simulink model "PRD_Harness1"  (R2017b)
settings: Solver=FixedStepDiscrete  StartTime=0.0  StopTime=4  FixedStep=0.01  RelTol=1e-3  EnableMultiTasking=on
undefined symbols (not defined in the file): sigbuilder_block

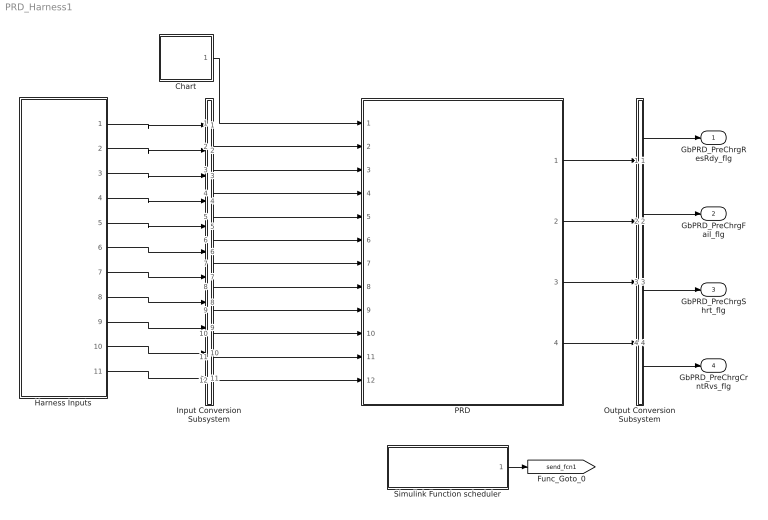
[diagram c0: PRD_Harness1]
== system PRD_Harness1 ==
  Chart : Stateflow chart  TreatAsAtomicUnit=on
  Harness Inputs : Subsystem  Tag=STV Subsys  LoadFcn=sigbuilder_block('load');  StartFcn=sigbuilder_block('start');  StopFcn=sigbuilder_block('stop');  ClipboardFcn=sigbuilder_block('clipboard');  mask(Sigbuilder block){tuvar=[0:10]}
      mask init:
      | if ~strcmp(get_param(bdroot(gcb),'SimulationStatus'),'stopped'),tuvar = sigbuilder_block('maskInit'); end
  Input Conversion Subsystem : Subsystem  Tag=__SLT_ICS__  Description=Signal spec. and routing
  Output Conversion Subsystem : Subsystem  Tag=__SLT_OCS__  Description=Signal spec. and routing
  PRD : ModelReference  ModelNameDialog=PRD  SimulationMode=Normal  ModelReferenceVersion='M101C101R103'
  Simulink Function scheduler : Test Sequence  Tag=__SLT_FCN_CALL__  TreatAsAtomicUnit=on
  GbPRD_PreChrgResRdy_flg : Outport  OutDataTypeStr=boolean  PortDimensions=[1]
  GbPRD_PreChrgFail_flg : Outport  Port=2  OutDataTypeStr=boolean  PortDimensions=[1]
  GbPRD_PreChrgShrt_flg : Outport  Port=3  OutDataTypeStr=boolean  PortDimensions=[1]
  GbPRD_PreChrgCrntRvs_flg : Outport  Port=4  OutDataTypeStr=boolean  PortDimensions=[1]
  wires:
  Harness Inputs/1(GeCTC_CtrCtlState_enum) -> Input Conversion Subsystem/1(Inport_1)
  Harness Inputs/2(GbCTC_PreChrgTimeOutFlt_flg) -> Input Conversion Subsystem/2(Inport_2)
  Harness Inputs/3(GcHDP_PackCrnt_A) -> Input Conversion Subsystem/3(Inport_3)
  Harness Inputs/4(GbHDP_PackCrntVld_flg) -> Input Conversion Subsystem/4(Inport_4)
  Harness Inputs/5(GbHDP_PackVoltVld_flg) -> Input Conversion Subsystem/5(Inport_5)
  Harness Inputs/6(GcHDP_PackVolt_V) -> Input Conversion Subsystem/6(Inport_6)
  Harness Inputs/7(GcHDP_PosCtlVolt_V) -> Input Conversion Subsystem/7(Inport_7)
  Harness Inputs/8(GbHDP_PosCtlVoltVld_flg) -> Input Conversion Subsystem/8(Inport_8)
  Harness Inputs/9(GcCDP_SumCellVolt_V) -> Input Conversion Subsystem/9(Inport_9)
  Harness Inputs/10(GbCDP_SumCellVoltVld_flg) -> Input Conversion Subsystem/10(Inport_10)
  Harness Inputs/11(GcRTC_ShelveTime_min) -> Input Conversion Subsystem/11(Inport_11)
  Output Conversion Subsystem/1(Outport_1) -> GbPRD_PreChrgResRdy_flg/1
  Output Conversion Subsystem/2(Outport_2) -> GbPRD_PreChrgFail_flg/1
  Output Conversion Subsystem/3(Outport_3) -> GbPRD_PreChrgShrt_flg/1
  Output Conversion Subsystem/4(Outport_4) -> GbPRD_PreChrgCrntRvs_flg/1
  Chart/1(RUN10ms()) -> PRD/1
  Input Conversion Subsystem/2(Outport_2) -> PRD/2
  Input Conversion Subsystem/3(Outport_3) -> PRD/3
  Input Conversion Subsystem/4(Outport_4) -> PRD/4
  Input Conversion Subsystem/5(Outport_5) -> PRD/5
  Input Conversion Subsystem/6(Outport_6) -> PRD/6
  Input Conversion Subsystem/7(Outport_7) -> PRD/7
  Input Conversion Subsystem/8(Outport_8) -> PRD/8
  Input Conversion Subsystem/9(Outport_9) -> PRD/9
  Input Conversion Subsystem/10(Outport_10) -> PRD/10
  Input Conversion Subsystem/11(Outport_11) -> PRD/11
  Input Conversion Subsystem/12(Outport_12) -> PRD/12
  PRD/1 -> Output Conversion Subsystem/1(Inport_1)
  PRD/2 -> Output Conversion Subsystem/2(Inport_2)
  PRD/3 -> Output Conversion Subsystem/3(Inport_3)
  PRD/4 -> Output Conversion Subsystem/4(Inport_4)
  Simulink Function scheduler/1(PRD_PreChrgResDiag_10ms()) -> [send_fcn1]

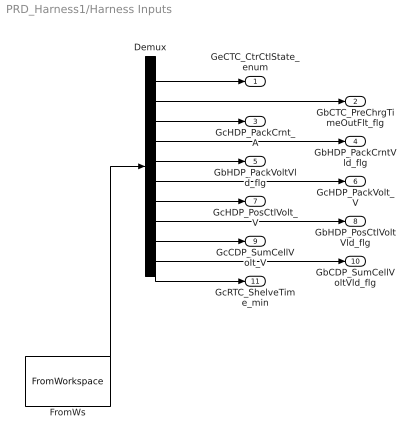
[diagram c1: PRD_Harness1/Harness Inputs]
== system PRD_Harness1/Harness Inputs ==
  Demux : Demux  Tag=STV Demux  Outputs=11
  FromWs : FromWorkspace  Tag=STV FromWs  VariableName=tuvar  SampleTime=0
  GeCTC_CtrCtlState_enum : Outport  Tag=STV Outport
  GbCTC_PreChrgTimeOutFlt_flg : Outport  Tag=STV Outport  Port=2
  GcHDP_PackCrnt_A : Outport  Tag=STV Outport  Port=3
  GbHDP_PackCrntVld_flg : Outport  Tag=STV Outport  Port=4
  GbHDP_PackVoltVld_flg : Outport  Tag=STV Outport  Port=5
  GcHDP_PackVolt_V : Outport  Tag=STV Outport  Port=6
  GcHDP_PosCtlVolt_V : Outport  Tag=STV Outport  Port=7
  GbHDP_PosCtlVoltVld_flg : Outport  Tag=STV Outport  Port=8
  GcCDP_SumCellVolt_V : Outport  Tag=STV Outport  Port=9
  GbCDP_SumCellVoltVld_flg : Outport  Tag=STV Outport  Port=10
  GcRTC_ShelveTime_min : Outport  Tag=STV Outport  Port=11
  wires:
  FromWs/1 -> Demux/1
  Demux/1 -> GeCTC_CtrCtlState_enum/1
  Demux/2 -> GbCTC_PreChrgTimeOutFlt_flg/1
  Demux/3 -> GcHDP_PackCrnt_A/1
  Demux/4 -> GbHDP_PackCrntVld_flg/1
  Demux/5 -> GbHDP_PackVoltVld_flg/1
  Demux/6 -> GcHDP_PackVolt_V/1
  Demux/7 -> GcHDP_PosCtlVolt_V/1
  Demux/8 -> GbHDP_PosCtlVoltVld_flg/1
  Demux/9 -> GcCDP_SumCellVolt_V/1
  Demux/10 -> GbCDP_SumCellVoltVld_flg/1
  Demux/11 -> GcRTC_ShelveTime_min/1

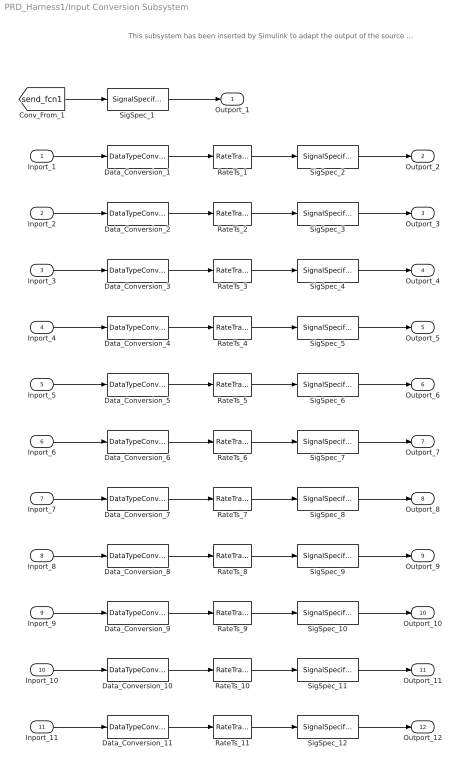
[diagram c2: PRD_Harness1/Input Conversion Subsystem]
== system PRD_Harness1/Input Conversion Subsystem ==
  note: This subsystem has been inserted by Simulink to adapt the output of the source blocks to the interface required by the harnessed component. Modifying the contents of this subsystem may result in compilation and simulation failure.
  Inport_1 : Inport
  Inport_2 : Inport  Port=2
  Inport_3 : Inport  Port=3
  Inport_4 : Inport  Port=4
  Inport_5 : Inport  Port=5
  Inport_6 : Inport  Port=6
  Inport_7 : Inport  Port=7
  Inport_8 : Inport  Port=8
  Inport_9 : Inport  Port=9
  Inport_10 : Inport  Port=10
  Inport_11 : Inport  Port=11
  Data_Conversion_1 : DataTypeConversion  OutDataTypeStr=uint8
  Data_Conversion_{2,4..5,8,10} (5 alike) : DataTypeConversion  OutDataTypeStr=boolean
  Data_Conversion_11 : DataTypeConversion  OutDataTypeStr=uint32
  Data_Conversion_{3,6..7,9} (4 alike) : DataTypeConversion  OutDataTypeStr=single
  RateTs_{1..11} (11 alike) : RateTransition
  SigSpec_1 : SignalSpecification
  SigSpec_10 : SignalSpecification  OutDataTypeStr=single  Unit=V  Dimensions=[1]
  SigSpec_{3,5..6,9,11} (5 alike) : SignalSpecification  OutDataTypeStr=boolean  Unit=flag  Dimensions=[1]
  SigSpec_12 : SignalSpecification  OutDataTypeStr=uint32  Unit=min  Dimensions=[1]
  SigSpec_2 : SignalSpecification  OutDataTypeStr=uint8  Unit=enum  Dimensions=[1]
  SigSpec_4 : SignalSpecification  OutDataTypeStr=single  Unit=A  Dimensions=[1]
  SigSpec_7 : SignalSpecification  OutDataTypeStr=single  Unit=V  Dimensions=[1]
  SigSpec_8 : SignalSpecification  OutDataTypeStr=single  Unit=V  Dimensions=[1]
  Outport_1 : Outport
  Outport_2 : Outport  Port=2
  Outport_3 : Outport  Port=3
  Outport_4 : Outport  Port=4
  Outport_5 : Outport  Port=5
  Outport_6 : Outport  Port=6
  Outport_7 : Outport  Port=7
  Outport_8 : Outport  Port=8
  Outport_9 : Outport  Port=9
  Outport_10 : Outport  Port=10
  Outport_11 : Outport  Port=11
  Outport_12 : Outport  Port=12
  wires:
  SigSpec_1/1 -> Outport_1/1
  [send_fcn1] -> SigSpec_1/1
  SigSpec_2/1 -> Outport_2/1
  RateTs_1/1 -> SigSpec_2/1
  Data_Conversion_1/1 -> RateTs_1/1
  Inport_1/1 -> Data_Conversion_1/1
  SigSpec_3/1 -> Outport_3/1
  RateTs_2/1 -> SigSpec_3/1
  Data_Conversion_2/1 -> RateTs_2/1
  Inport_2/1 -> Data_Conversion_2/1
  SigSpec_4/1 -> Outport_4/1
  RateTs_3/1 -> SigSpec_4/1
  Data_Conversion_3/1 -> RateTs_3/1
  Inport_3/1 -> Data_Conversion_3/1
  SigSpec_5/1 -> Outport_5/1
  RateTs_4/1 -> SigSpec_5/1
  Data_Conversion_4/1 -> RateTs_4/1
  Inport_4/1 -> Data_Conversion_4/1
  SigSpec_6/1 -> Outport_6/1
  RateTs_5/1 -> SigSpec_6/1
  Data_Conversion_5/1 -> RateTs_5/1
  Inport_5/1 -> Data_Conversion_5/1
  SigSpec_7/1 -> Outport_7/1
  RateTs_6/1 -> SigSpec_7/1
  Data_Conversion_6/1 -> RateTs_6/1
  Inport_6/1 -> Data_Conversion_6/1
  SigSpec_8/1 -> Outport_8/1
  RateTs_7/1 -> SigSpec_8/1
  Data_Conversion_7/1 -> RateTs_7/1
  Inport_7/1 -> Data_Conversion_7/1
  SigSpec_9/1 -> Outport_9/1
  RateTs_8/1 -> SigSpec_9/1
  Data_Conversion_8/1 -> RateTs_8/1
  Inport_8/1 -> Data_Conversion_8/1
  SigSpec_10/1 -> Outport_10/1
  RateTs_9/1 -> SigSpec_10/1
  Data_Conversion_9/1 -> RateTs_9/1
  Inport_9/1 -> Data_Conversion_9/1
  SigSpec_11/1 -> Outport_11/1
  RateTs_10/1 -> SigSpec_11/1
  Data_Conversion_10/1 -> RateTs_10/1
  Inport_10/1 -> Data_Conversion_10/1
  SigSpec_12/1 -> Outport_12/1
  RateTs_11/1 -> SigSpec_12/1
  Data_Conversion_11/1 -> RateTs_11/1
  Inport_11/1 -> Data_Conversion_11/1

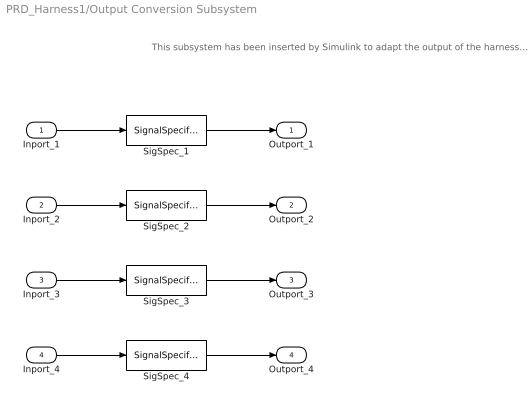
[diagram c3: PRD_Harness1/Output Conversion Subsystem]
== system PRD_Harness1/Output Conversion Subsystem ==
  note: This subsystem has been inserted by Simulink to adapt the output of the harnessed component to the interface required by the sink blocks. Modifying the contents of this subsystem may result in compilation and simulation failure.
  Inport_1 : Inport
  Inport_2 : Inport  Port=2
  Inport_3 : Inport  Port=3
  Inport_4 : Inport  Port=4
  SigSpec_{1..4} (4 alike) : SignalSpecification  OutDataTypeStr=boolean  Unit=flag  Dimensions=[1]
  Outport_1 : Outport
  Outport_2 : Outport  Port=2
  Outport_3 : Outport  Port=3
  Outport_4 : Outport  Port=4
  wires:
  Inport_1/1 -> SigSpec_1/1
  SigSpec_1/1 -> Outport_1/1
  Inport_2/1 -> SigSpec_2/1
  SigSpec_2/1 -> Outport_2/1
  Inport_3/1 -> SigSpec_3/1
  SigSpec_3/1 -> Outport_3/1
  Inport_4/1 -> SigSpec_4/1
  SigSpec_4/1 -> Outport_4/1

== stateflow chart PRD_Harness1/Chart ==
  (default) -> (junction 1)
  (junction 1) -> (junction 3) : {RUN10ms}
  events: output FUNCTION_CALL_EVENT

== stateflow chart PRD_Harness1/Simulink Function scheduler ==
  state Run
  state AsyncFunctionCalls
    % Call Asynchronous FunctionCall Subsystems.
    %
    %% Schedule function-call outputs.
    %% Modify this code to change function-call order.
    send(PRD_PreChrgResDiag_10ms)
  (default) -> Run
  events: output FUNCTION_CALL_EVENT
